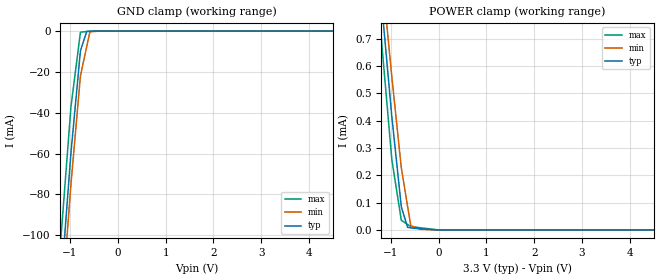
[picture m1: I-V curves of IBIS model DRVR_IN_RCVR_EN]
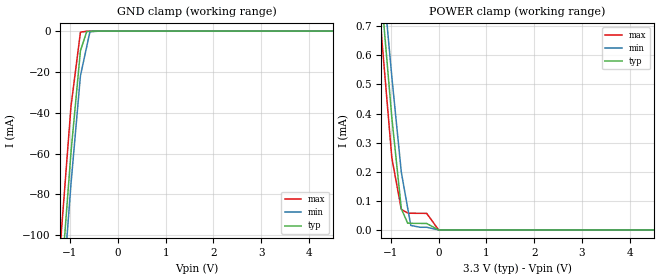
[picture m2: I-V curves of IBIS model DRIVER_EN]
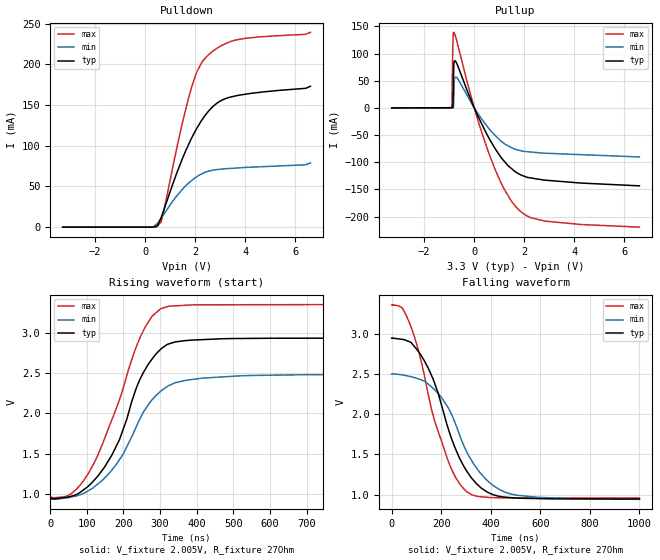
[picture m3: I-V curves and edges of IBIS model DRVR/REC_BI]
|Texas Instruments Incorporated
|3.3V RS-485 Transceivers
|Models valid upto 1Mbps Signaling Rate
| Marketing part#   Voltage Range   Package-type   #pins/pkg drawing
|SN65HVD12DR   3.0V to 3.6V   SOIC   8-pin D
|SN65HVD12DRG4   3.0V to 3.6V   SOIC   8-pin D
|SN65HVD12DG4   3.0V to 3.6V   SOIC   8-pin D
|SN65HVD12D   3.0V to 3.6V   SOIC   8-pin D
|SN65HVD12P   3.0V to 3.6V   PDIP   8-pin P
|SN65HVD12PE4   3.0V to 3.6V   PDIP   8-pin P
[IBIS Ver]   4.0
[File name]   sn65hvd12.ibs
[File Rev]   2.0
[Date]   02/03/2010
[Source]   TISPICED simulations at:
   Texas Instruments Incorporated.
   Analog-eLab, HPA
   12500 TI Blvd
   Dallas, TX -75243
   For Support e-mail: elab_ibis@list.ti.com
[Notes]   Revision History:
   Rev 1.2: 11/18/2009
   - Initial Version originated by Data Transmission Products Group
   Rev 2.0: 02/03/2010
   - Updated all models to match latest simulations in TISPICED
   - Ignore warnings related ccomp; the numbers are based on simulation
   PVT conditions
   - Non-monotonic warnings are related to pullup is inherent to buffer
   structure
[Disclaimer]
 This product is designed as an aid for customers of Texas Instruments.
 No warranties, either expressed or implied, with respect to this third
 party software (if any) or with respect to its fitness for any
 particular purpose is claimed by Texas Instruments or the author. The
 software (if any) is provided solely on an "as is" basis. The entire
 risk as to its quality and performance is with the customer
[Copyright] (C) Copyright 2010 Texas Instruments Incorporated.
   All rights reserved.
|   SN65HVD12D SOIC 8-pin D package
[Component]   SN65HVD12D
[Manufacturer]  Texas Instruments Incorporated
[Package]   |SOIC 8-pin D package
|   typ   min   max
R_pkg   0.0679   0.0575   0.0785
L_pkg   2.53609nH   2.2863nH   2.7859nH
C_pkg   0.39065pF   0.3817pF   0.3996pF
[Pin]   signal_name   model_name   R_pin   L_pin   C_pin
1   R   RECEIVER_OUT   0.07682  2.75302nH  0.38833pF
2   RE   DRVR_IN_RCVR_EN   0.06188  2.38320nH  0.38653pF
3   DE   DRIVER_EN   0.07494  2.65996nH  0.39957pF
4   D   DRVR_IN_RCVR_EN   0.07845  2.78591nH  0.38888pF
5   GND   GND   0.03332  2.17766nH  0.40720pF
6   A   DRVR/REC_BI   0.05760  2.29746nH  0.38353pF
7   B   DRVR/REC_BI   0.05748  2.28626nH  0.38173pF
8   VCC   POWER   0.03357  2.17742nH  0.40796pF
[Diff_pin]   inv_pin   vdiff   tdelay_typ   tdelay_min   tdelay_max
| The 'A' pin is Diff_pin and the 'B' pin is the inv_pin
6   7   0.200   0 0 0
| Models and submodels in the file (4): DRVR_IN_RCVR_EN (Input), DRIVER_EN (Input), DRVR/REC_BI (I/O), RECEIVER_OUT (Output)
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|   Driver Input / Receiver Enable Model
[Model]   DRVR_IN_RCVR_EN
Model_type   Input
|Signals   D,RE
Vinl = 0.8V
Vinh = 2V
|   typ   min   max
C_comp   7.89pF   8.31pF   7.55pF
[Voltage Range]   3.3V   3V   3.6V
[Temperature Range]   25   85   -40
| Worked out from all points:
|   GND clamp passes 1 mA (typ) near -0.66 V on its own axis
|   POWER clamp passes 1 mA (typ) near -1.28 V on its own axis
[GND Clamp]
|   Voltage   I(typ)   I(min)   I(max)
-3.3V     -813.9mA   -834.3mA   -783.4mA
-1.178V   -120.8mA   -136.3mA   -97.45mA
-979.8mV  -59.48mA   -74.9mA    -37.01mA
-781.8mV  -9.63mA    -21.9mA    -533.6uA
-650.4mV  -211.5uA   -7.61mA    -205.7uA
-583.8mV  -112.9uA   -367.2uA   -39.42uA
-385.8mV  -14.39uA   -9.036uA   -34.36uA
6.6V      0A         0A         0A
[POWER Clamp]
|   Voltage   I(typ)   I(min)   I(max)
-3.3V     5.197mA    4.974mA    5.426mA
-1.376V   1.195mA    1.285mA    1.083mA
-1.178V   797.1uA    917.4uA    654.7uA
-979.8mV  413.4uA    559.5uA    256.9uA
-781.8mV  84.75uA    226.8uA    35.24uA
-650.4mV  9.528uA    86.78uA    20.15uA
-583.8mV  7.807uA    15.82uA    12.5uA
-385.8mV  4.52uA     2.606uA    8.214uA
0V        0A         0A         0A
6.6V      0A         0A         0A
|   Driver Enable Model
[Model]   DRIVER_EN
Model_type   Input
|Signals   DE
Vinl = 0.8V
Vinh = 2V
|   typ   min   max
C_comp   7.89pF   8.31pF   7.55pF
[Voltage Range]   3.3V   3V   3.6V
[Temperature Range]   25   85   -40
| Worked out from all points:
|   GND clamp passes 1 mA (typ) near -0.66 V on its own axis
|   POWER clamp passes 1 mA (typ) near -1.29 V on its own axis
[GND Clamp]
|   Voltage   I(typ)   I(min)   I(max)
-3.3V     -813.9mA   -834.3mA   -783.3mA
-1.178V   -120.8mA   -136.3mA   -97.42mA
-979.8mV  -59.48mA   -74.9mA    -36.99mA
-781.8mV  -9.629mA   -21.9mA    -539.3uA
-649.7mV  -208.6uA   -7.538mA   -75.09uA
-583.8mV  -112.4uA   -371.3uA   -34.61uA
-385.8mV  -9.744uA   -8.088uA   -20.64uA
6.6V      0A         0A         0A
[POWER Clamp]
|   Voltage   I(typ)   I(min)   I(max)
-3.3V     5.163mA    4.937mA    5.398mA
-1.376V   1.163mA    1.249mA    1.058mA
-1.178V   766.2uA    882.2uA    632.6uA
-979.8mV  385.3uA    525.8uA    247.6uA
-781.8mV  73.21uA    198.5uA    70.5uA
-649.7mV  23.45uA    76.53uA    58.57uA
-583.8mV  23.05uA    15.68uA    57.53uA
-385.8mV  22.6uA     9.295uA    57.26uA
-251.7mV  22.43uA    9.265uA    57.15uA
0V        0A         0A         0A
6.6V      0A         0A         0A
|   Driver Output / Receiver Input Model
[Model]   DRVR/REC_BI
Model_type   I/O
Polarity   Non-Inverting
Enable   Active-High
| Signals   A,B
Vinl = 0.9V
Vinh = 2.8V
Vmeas = 2.005V   |Reference voltage for timing measurements
Cref = 15pF   |Timing specification test load capacitance value
Rref = 27   |Note: 54 Ohm load; single-ended configuration
Vref= 2.005V
|   Timing specification test load voltage
| variable   typ   min   max
|C_comp Driver off/RCV enabled
C_comp   47.166pF   47.286pF   47.970pF
|C_comp (Output HIGH state)66.728pF   66.338pF   68.991pF
|C_comp (Output LOW state) 66.735pF   66.339pF   69.006pF
|   typ   min   max
[Temperature Range]   25.0   85.0   -40
[Voltage range]   3.3V   3.0V   3.6V
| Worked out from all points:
|   slope of the pulldown table from 0 to 0.495 V, typ, clamps not added: 228 ohm
|   slope of the pullup table from 0 to 0.495 V, typ, clamps not added: 10.4 ohm
|   falling waveform, V_fixture 2.005V, R_fixture 27Ohm: 20-80 % time 141ns typ, 157ns min, 126ns max; typ from 2.95 V to 0.945 V
|   rising waveform, V_fixture 2.005V, R_fixture 27Ohm: 20-80 % time 109ns typ, 121ns min, 114ns max; typ from 0.945 V to 2.93 V
[Pulldown]
|   Voltage   I(typ)   I(min)   I(max)
-3.3V     -10.36nA   -11.51nA   -9.421nA
176.9mV   1.608uA    4.179uA    2.728uA
437.7mV   1.189mA    3.334mA    2.934uA
485.7mV   1.569mA    4.55mA     1.475mA
635.7mV   11.65mA    11.05mA    6.077mA
1.412V    78.41mA    43.8mA     118.2mA
1.877V    110.8mA    57.83mA    174.4mA
2.068V    121.8mA    62.11mA    191.3mA
2.315V    133.8mA    66.22mA    204.6mA
2.85V     151.8mA    70.6mA     219.3mA
3.382V    159.5mA    72.07mA    227.5mA
6.6V      173mA      78.91mA    239.2mA
[GND Clamp]
|   Voltage   I(typ)   I(min)   I(max)
-3.3V     0A         0A         0A
0V        0A         0A         0A
6.6V      0A         0A         0A
[Pullup]
|   Voltage   I(typ)   I(min)   I(max)
-3.3V     11.44nA    9.077nA    13.92nA
-905.4mV  445.9uA    311.3uA    528.4uA
-894.5mV  447.9uA    312.7uA    5.965mA
-854.4mV  3.819mA    317.9uA    116.8mA
-818.1mV  76.91mA    19.7mA     139.1mA
-790.6mV  86.17mA    54.02mA    137.1mA
-705.4mV  82.38mA    56.14mA    124.1mA
-27.68mV  3.039mA    2.124mA    4.49mA
635.7mV   -59.56mA   -40.88mA   -90.04mA
1.718V    -119.7mA   -77.18mA   -184.7mA
2.812V    -132.8mA   -83.25mA   -207.9mA
6.6V      -143.3mA   -90.21mA   -219.3mA
[POWER Clamp]
|   Voltage   I(typ)   I(min)   I(max)
-3.3V     0A         0A         0A
0V        0A         0A         0A
6.6V      0A         0A         0A
[Ramp]
R_load = 27
|   typ   min   max
dV/dt_r   1.19342/1.08688e-007  0.926663/1.20451e-007   1.43664/1.14095e-007
dV/dt_f   1.20198/1.40835e-007  0.936588/1.56597e-007   1.44283/1.25896e-007
[Falling Waveform]
V_fixture = 2.005V
V_fixture_min = 1.616V
V_fixture_max = 2.362V
R_fixture = 27Ohm
C_fixture = 0F
|   Time   V(typ)   V(min)   V(max)
0s        2.948V     2.501V     3.361V
57.35ns   2.922V     2.482V     3.241V
93.66ns   2.838V     2.455V     2.947V
130.8ns   2.673V     2.414V     2.501V
174.4ns   2.377V     2.302V     1.905V
226.1ns   1.842V     2.092V     1.436V
301ns     1.301V     1.546V     1.039V
383.2ns   1.036V     1.182V     966.3mV
478.6ns   962mV      1.009V     958.2mV
1us       944.6mV    940.4mV    956.4mV
[Rising Waveform]
V_fixture = 2.005V
V_fixture_min = 1.616V
V_fixture_max = 2.362V
R_fixture = 27Ohm
C_fixture = 0F
|   Time   V(typ)   V(min)   V(max)
0s        944.6mV    939.2mV    956.4mV
72.29ns   998.8mV    979.7mV    1.066V
105.9ns   1.108V     1.048V     1.272V
147.6ns   1.332V     1.196V     1.681V
188.7ns   1.672V     1.425V     2.165V
246.5ns   2.436V     1.948V     2.954V
277.9ns   2.674V     2.168V     3.204V
301ns     2.794V     2.273V     3.297V
416.6ns   2.916V     2.438V     3.347V
1us       2.934V     2.484V     3.351V
